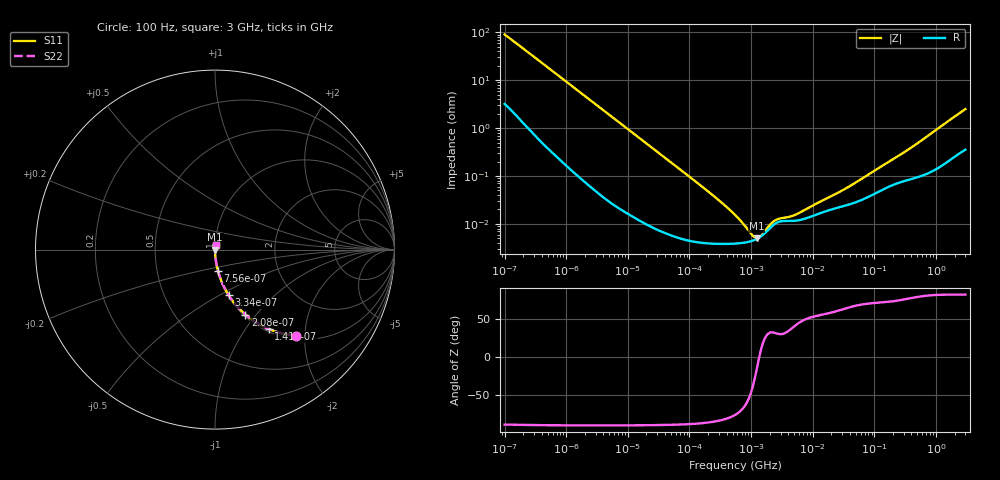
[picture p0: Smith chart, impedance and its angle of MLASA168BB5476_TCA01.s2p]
! MLASA168BB5476_TCA01  S-PARAMETER MODEL  ( Standard Model )
! Model Generated by TAIYO YUDEN Corporation (http://www.ty-top.com)
! Version 1.0
! TAIYO YUDEN Control No. 241206
! Copyright(c) 2024 TAIYO YUDEN CO.,LTD. All Rights Reserved.
! Product Description (link to TY-COMPAS)
! https://ds.yuden.co.jp/TYCOMPAS/or/detail?pn=MLASA168BB5476MTCA01&u=M
! Products Name : Multilayer Ceramic Capacitors
! Characteristics :
!  Capacitance : 47 [uF] , Rated Voltage : 4 [V] , TCC : X5R
!  Case Size : 1.6 x 0.8 / 0.063 x 0.031 [mm/inch] , Thickness : 0.8 / 0.031 [mm/inch]
!  (Conditions: Temperature = 25 [degC] , DC Bias Voltage = 0 [V])
! External Node Assignments :
!  1  o---| |---o  2
! GND o---------o GND
! Frequency Range : 100Hz  -  3GHz  [ 401 STEP ]
# MHZ S RI R 50
! Freq[MHz].  S11 Real  S11 Imag  S21 Real  S21 Imag  S12 Real  S12 Imag  S22 Real  S22 Imag
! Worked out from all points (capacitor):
!   401 points, 100 Hz to 3 GHz, reference 50 ohm
!   read as one part in series: C = 17.5 uF near 109 Hz
!   lowest |Z| = 5.03 mohm at 1.241 MHz (marker M1)
!   series resonance near 1.353 MHz, so ESL is about 790 pH
!   S11 on the Smith chart (normalised r, x): 100 Hz: 1.06, -1.80; 141 Hz: 1.04, -1.29; 208 Hz: 1.02, -0.88; 334 Hz: 1.01, -0.55; 756 Hz: 1.00, -0.25; 3 GHz: 1.01, +0.05
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0.0001  0.4502 -0.4801  0.5498 0.4801  0.5498 0.4801  0.4502 -0.4801
0.000141  0.2998 -0.4424  0.7002 0.4424  0.7002 0.4424  0.2998 -0.4424
0.000208  0.1698 -0.362  0.8302 0.362  0.8302 0.362  0.1698 -0.362
0.000334  0.0761 -0.254  0.9239 0.254  0.9239 0.254  0.0761 -0.254
0.000756  0.0171 -0.1208  0.9829 0.1208  0.9829 0.1208  0.0171 -0.1208
0.001788  0.00359 -0.0523  0.9964 0.0523  0.9964 0.0523  0.00359 -0.0523
0.005476  0.000565 -0.0173  0.9994 0.0173  0.9994 0.0173  0.000565 -0.0173
0.031977  8.17e-05 -0.00301  0.9999 0.00301  0.9999 0.00301  8.17e-05 -0.00301
0.221826  3.9e-05 -0.000427  1 0.000427  1 0.000427  3.9e-05 -0.000427
0.547723  3.88e-05 -0.00015  1 0.00015  1 0.00015  3.88e-05 -0.00015
0.709116  4e-05 -0.000101  1 0.000101  1 0.000101  4e-05 -0.000101
0.772864  4.06e-05 -8.59e-05  1 8.59e-05  1 8.59e-05  4.06e-05 -8.59e-05
1.240863  4.87e-05 -1.26e-05  1 1.26e-05  1 1.26e-05  4.87e-05 -1.26e-05
1.992254  7.97e-05 4.95e-05  0.9999 -4.95e-05  0.9999 -4.95e-05  7.97e-05 4.95e-05
2.81117  0.000111 6.47e-05  0.9999 -6.47e-05  0.9999 -6.47e-05  0.000111 6.47e-05
5.135543  0.000116 0.000101  0.9999 -0.000101  0.9999 -0.000101  0.000116 0.000101
9.794414  0.000145 0.000189  0.9999 -0.000189  0.9999 -0.000189  0.000145 0.000189
35.62563  0.000246 0.000507  0.9998 -0.000507  0.9998 -0.000507  0.000246 0.000507
175.1444  0.000609 0.00191  0.9994 -0.00191  0.9994 -0.00191  0.000609 0.00191
414.2403  0.000892 0.00397  0.9991 -0.00397  0.9991 -0.00397  0.000892 0.00397
1950.712  0.00273 0.0167  0.9973 -0.0167  0.9973 -0.0167  0.00273 0.0167
3000  0.00413 0.0245  0.9959 -0.0245  0.9959 -0.0245  0.00413 0.0245
